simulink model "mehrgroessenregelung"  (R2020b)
settings: Solver=VariableStepAuto  StartTime=0.0  StopTime=60  RelTol=1e-3
model workspace (MAT data in the model file):
  K_IR1 = 1.25
  K_IR2 = 0.42
  K_P11 = 0.2
  K_P12 = 0.2
  K_P21 = 0.1
  K_P22 = 0.4
  T_11 = 2
  T_22 = 3

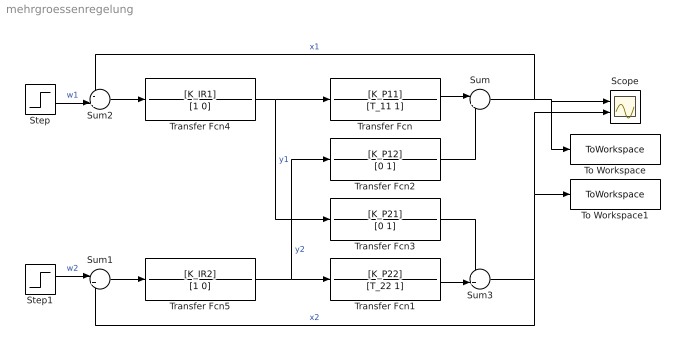
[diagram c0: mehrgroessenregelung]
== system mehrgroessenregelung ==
  Scope : Scope  NumInputPorts=2
  Step : Step  Time=3  SampleTime=0
  Step1 : Step  Time=30  After=-0.5  SampleTime=0
  Sum : Sum  Inputs=|++
  Sum1 : Sum  Inputs=|+-
  Sum2 : Sum  Inputs=-+|
  Sum3 : Sum  Inputs=++|
  To Workspace : ToWorkspace  VariableName=x1  SaveFormat=Timeseries  SampleTime=-1
  To Workspace1 : ToWorkspace  VariableName=x2  SaveFormat=Timeseries  SampleTime=-1
  Transfer Fcn : TransferFcn  Numerator=[K_P11]  Denominator=[T_11 1]
  Transfer Fcn1 : TransferFcn  Numerator=[K_P22]  Denominator=[T_22 1]
  Transfer Fcn2 : TransferFcn  Numerator=[K_P12]  Denominator=[0 1]
  Transfer Fcn3 : TransferFcn  Numerator=[K_P21]  Denominator=[0 1]
  Transfer Fcn4 : TransferFcn  Numerator=[K_IR1]  Denominator=[1 0]
  Transfer Fcn5 : TransferFcn  Numerator=[K_IR2]  Denominator=[1 0]
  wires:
  Transfer Fcn/1 -> Sum/1
  Transfer Fcn2/1 -> Sum/2
  Transfer Fcn4/1 -> Transfer Fcn3/1, Transfer Fcn/1  "y1"
  Sum2/1 -> Transfer Fcn4/1
  Sum/1 -> Sum2/1, To Workspace/1, Scope/1  "x1"
  Step/1 -> Sum2/2  "w1"
  Transfer Fcn5/1 -> Transfer Fcn2/1, Transfer Fcn1/1  "y2"
  Sum1/1 -> Transfer Fcn5/1
  Step1/1 -> Sum1/1  "w2"
  Transfer Fcn1/1 -> Sum3/2
  Transfer Fcn3/1 -> Sum3/1
  Sum3/1 -> To Workspace1/1, Scope/2, Sum1/2  "x2"
